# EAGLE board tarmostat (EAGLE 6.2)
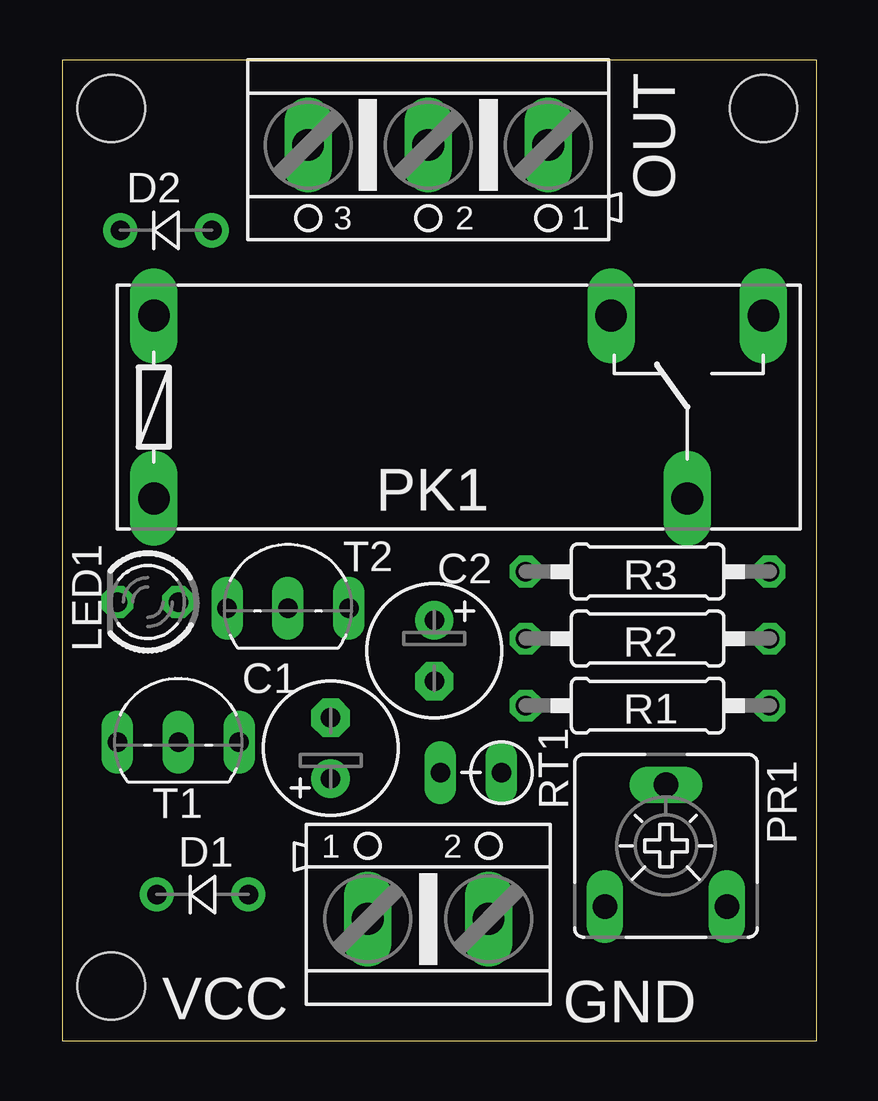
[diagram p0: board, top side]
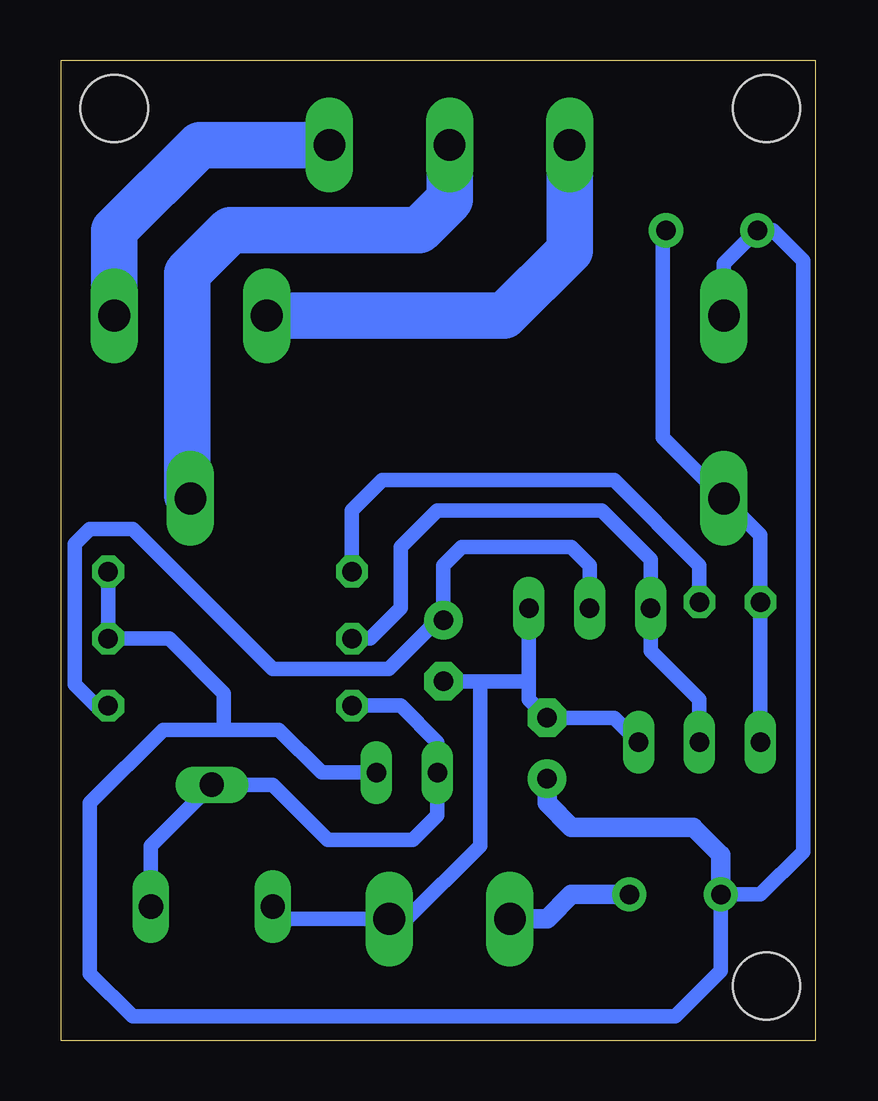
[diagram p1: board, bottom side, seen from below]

Size 31.42 x 40.88 mm. Coordinates in mm from the lower left corner, seen from the top.
Outline: 0,0 31.42,0 31.42,40.88 0,40.88 0,0
Copper layers (1*16): Top 0.035mm / dielectric 1.5mm / Bottom 0.035mm
Design rules: minimum track width 10mil, minimum drill 24mil, track to track 8mil, track to pad 8mil, pad to pad 8mil, via to via 8mil, smd to smd 8mil, copper to edge 40mil, drill to drill 8mil, minimum pad ring 10mil, minimum via ring 8mil, stop-mask expansion 4mil, vias tented up to drill 0mil, thermal gap 10mil
Holes 2.8 mm at 2.03,38.86 29.21,38.86 2.03,2.29

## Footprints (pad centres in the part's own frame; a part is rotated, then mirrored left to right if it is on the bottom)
E2,5-6 = drill 0.813 pad 1.6: + -1.27,0 | drill 0.813 pad 1.6 octagon: - 1.27,0
D-2.5 = drill 0.813 pad 1.422: A 1.905,0; C -1.905,0
LED3MM = drill 0.813 octagon: A -1.27,0; K 1.27,0
AK500/3 = drill 1.321 long: 1 -5.004,0; 2 0,0; 3 5.004,0
G6RW = drill 1.321 long: 1 -12.7,-3.81; 2 -12.7,3.81; O 6.35,3.81; P 9.525,-3.81; S 12.7,3.81
CA6V = drill 1.016 long: A -2.54,-2.54; E 2.54,-2.54; S 0,2.54
0207/10 = drill 0.813 octagon: 1 -5.08,0; 2 5.08,0
RS-2,5 = drill 0.813 long: 1 -1.27,0; 2 1.27,0
TO92-CBE = drill 0.813 long: B 0,0; C -2.54,0; E 2.54,0
AK500/2 = drill 1.321 long: 1 -2.515,0; 2 2.515,0

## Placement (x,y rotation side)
C1  [E2,5-6]  11.18,12.19 90 top
C2  [E2,5-6]  15.49,16.26 270 top
D1  [D-2.5]  5.84,6.1 0 top
D2  [D-2.5]  4.32,33.78 0 top
LED1  [LED3MM]  3.56,18.29 180 top
OUT  [AK500/3]  15.24,37.34 180 top
PK1  [G6RW]  16.51,26.42 0 top
PR1  10k  [CA6V]  25.15,8.13 0 top
R1  [0207/10]  24.38,13.97 180 top
R2  [0207/10]  24.38,16.76 180 top
R3  [0207/10]  24.38,19.56 0 top
RT1  10k  [RS-2,5]  17.02,11.18 180 top
T1  [TO92-CBE]  4.83,12.45 0 top
T2  [TO92-CBE]  9.4,18.03 0 top
VCC  [AK500/2]  15.24,5.08 0 top

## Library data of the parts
C1 C2 R1-R3 = rcl
D1 D2 = diode
LED1 = led
OUT VCC = con-ptr500; OC_FARNELL: unknown; OC_NEWARK: unknown
PK1 = relay; OC_FARNELL: unknown; OC_NEWARK: unknown
PR1 = pot
RT1 = varistor
T1 T2 = transistor

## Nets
N$1: C1.+ D1.C D2.C PK1.2 R2.1 R3.2 RT1.1
N$2: R2.2 T1.B T2.C
N$3: OUT.2 PK1.P
N$5: C1.- C2.- PR1.A T1.E T2.E VCC.2
N$6: LED1.A R3.1
N$7: D1.A VCC.1
N$9: C2.+ R1.1 T2.B
N$10: PR1.E PR1.S R1.2 RT1.2
N$11: D2.A LED1.K PK1.1 T1.C
N$14: OUT.3 PK1.O
N$16: OUT.1 PK1.S

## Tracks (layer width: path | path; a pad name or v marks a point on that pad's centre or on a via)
N$1
  Bottom 0.61: R3.2 R2.1 26.92,16.76 24.64,14.48 24.64,12.95 | RT1.1 20.57,11.18 22.35,12.95 24.64,12.95 | PK1.2 3.81,32.39 D2.C 1.78,33.78 0.51,32.51 0.51,7.87 2.29,6.1 D1.C 3.94,2.92 5.84,1.02 28.45,1.02 30.23,2.79 30.23,9.91 27.18,12.95 24.64,12.95
  Bottom 0.813: D1.C 3.94,7.75 5.08,8.89 10.16,8.89 11.18,9.91 C1.+
N$2
  Bottom 0.61: T1.B 4.83,14.22 6.86,16.26 T2.C 6.86,20.07 8.89,22.1 15.75,22.1 17.27,20.57 17.27,18.03 18.54,16.76 R2.2
N$3
  Bottom 1.422: 26.16,22.73 PK1.P
  Bottom 1.93: OUT.2 15.24,35.05 16.51,33.78 24.38,33.78 26.16,32 26.16,22.73
N$5
  Bottom 0.61: PR1.A 22.1,5.08 VCC.2 17.02,5.08 13.97,8.13 13.97,14.99 | T2.E 11.94,14.99 | 11.94,14.99 11.94,14.22 C1.- 8.38,13.46 T1.E | C2.- 13.97,14.99 | 13.97,14.99 11.94,14.99
N$6
  Bottom 0.61: R3.1 19.3,22.1 18.03,23.37 8.38,23.37 4.83,19.81 LED1.A
N$7
  Bottom 0.813: D1.A 10.16,6.1 11.18,5.08 VCC.1
N$9
  Bottom 0.61: R1.1 29.97,13.97 30.86,14.86 30.86,20.7 30.23,21.34 28.45,21.34 22.61,15.49 17.78,15.49 15.75,17.53 C2.+ 15.49,19.81 14.73,20.57 10.16,20.57 9.4,19.81 T2.B
N$10
  Bottom 0.61: PR1.E 27.69,8.13 PR1.S 22.61,10.67 20.32,8.38 16.76,8.38 15.75,9.4 RT1.2 15.75,12.45 17.27,13.97 R1.2
N$11
  Bottom 0.61: T1.C LED1.K 2.29,21.08 PK1.1 6.35,25.15 6.35,33.66 D2.A
N$14
  Bottom 1.93: OUT.3 10.24,32.94 12.95,30.23 PK1.O
N$16
  Bottom 1.93: PK1.S 29.21,33.78 25.65,37.34 OUT.1

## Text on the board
tNames: GND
